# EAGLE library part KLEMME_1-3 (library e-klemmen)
Klemme 3 Pol.
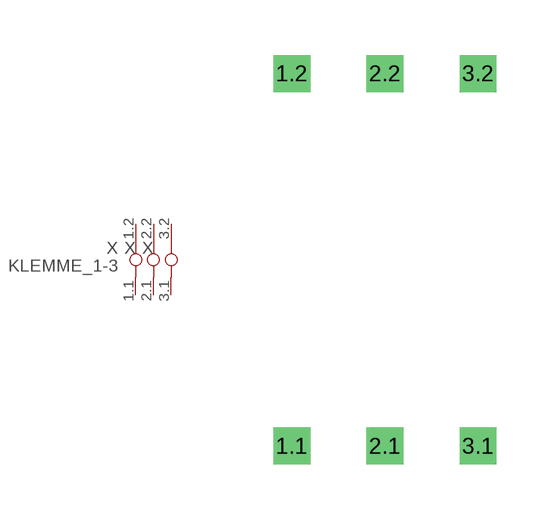
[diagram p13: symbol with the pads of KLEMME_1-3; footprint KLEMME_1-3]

Designator prefix X; gates 1=KLEMME_1-1 2=KLEMME_2 3=KLEMME_3

## KLEMME_1-3  [KLEMME_1-3]
1.1  1:1.1  pas
1.2  1:1.2  pas
2.1  2:2.1  pas
2.2  2:2.2  pas
3.1  3:3.1  pas
3.2  3:3.2  pas

## Footprint KLEMME_1-3 (pad centres in mm)
Dummy
drill 0.5 pad 1 square: 1.1 0,-12.7; 1.2 0,-2.54; 2.1 2.54,-12.7; 2.2 2.54,-2.54; 3.1 5.08,-12.7; 3.2 5.08,-2.54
